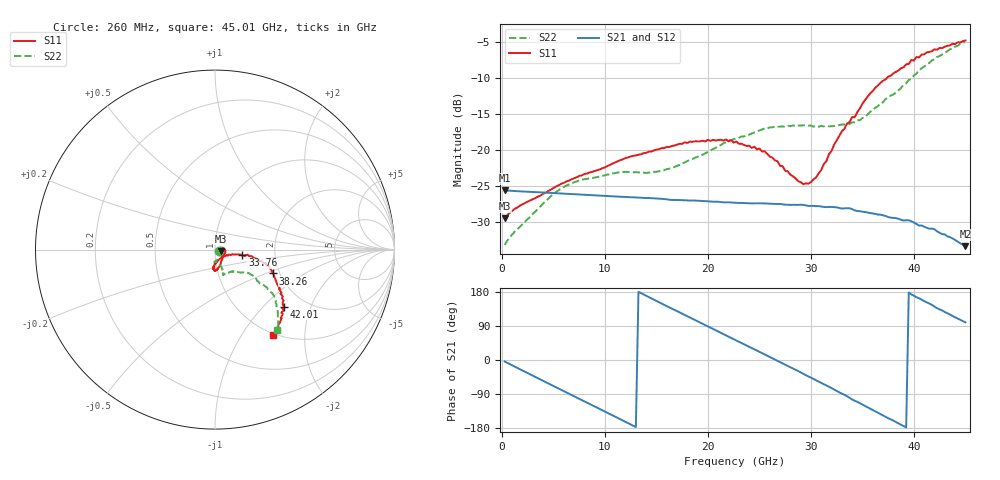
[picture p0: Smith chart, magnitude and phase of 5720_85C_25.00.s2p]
! Device:  ADRF5720
! Description: 0.5dB LSB GaAs MMIC 6-bit Digital Attenuator
! Frequency:  0.000009 -  40 GHz
! Ports:
!	RF1	= Port 1
!	RF2	= Port 2
! Vdd:  3.3 Volt
! Vss:  -3.3 Volt
! Control:  0/3.3 Volt
! State:  25.00 dB attenuation
! Data:  The device was measured using G-S-G Probes on a matrix board.
!  Data was collected using an calibrated 4 port network analyzer.
!  The reference plane for this measurement is at the launchers.
! Note:  Analog Devices supplies this data as a sample of measured data
!  for this product.  Your particular data for this product may vary.
!  Data was taken at 85 degrees C.
!  Analog Devices reserves the right to change this data at anytime.
# GHZ S DB R 45.0
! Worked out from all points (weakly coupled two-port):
!   180 points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, 260 MHz to 45.01 GHz, reference 45 ohm
!   highest |S21| = -25.66 dB at 260 MHz (marker M1); lowest = -33.4 dB at 45.01 GHz (marker M2)
!   lowest |S11| = -29.5 dB at 260 MHz (marker M3), VSWR 1.07, Z = 48 - j0.787 ohm
!   |S11| at or under -10 dB: start of sweep to 37.39 GHz
!   |S22| runs from -33.2 to -4.9 dB; largest |S21 - S12| = 0.00029
!   S11 on the Smith chart (normalised r, x): 260 MHz: 1.07, -0.02; 33.76 GHz: 1.36, -0.09; 38.26 GHz: 1.84, -0.56; 42.01 GHz: 1.57, -1.33; 45.01 GHz: 0.97, -1.39
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0.26  -29.52 -14.2  -25.66 -3.8  -25.66 -3.8  -33.25 -22.7
1.26  -28.21 -3.8  -25.75 -17.8  -25.74 -17.7  -31.37 -14.5
4.76  -25.54 -36.0  -26.01 -65.4  -26.00 -65.4  -26.45 -66.1
6.26  -24.41 -45.2  -26.13 -85.7  -26.12 -85.6  -24.98 -76.4
7.76  -23.57 -52.6  -26.25 -105.9  -26.24 -105.8  -24.19 -83.4
11.51  -21.44 -68.3  -26.55 -156.4  -26.54 -156.3  -23.11 -92.8
15.26  -19.92 -78.0  -26.80 152.4  -26.79 152.5  -22.99 -85.3
18.26  -18.86 -84.7  -27.07 112.2  -27.05 112.3  -21.42 -75.3
22.76  -18.86 -92.2  -27.38 51.5  -27.36 51.7  -18.44 -69.8
25.51  -20.21 -93.1  -27.47 14.8  -27.45 15.1  -17.04 -71.9
29.26  -24.78 -59.8  -27.67 -36.4  -27.65 -36.2  -16.60 -71.4
30.26  -24.12 -41.1  -27.81 -49.9  -27.79 -49.6  -16.79 -70.3
31.01  -22.83 -24.1  -27.90 -60.5  -27.88 -60.2  -16.67 -68.0
33.01  -17.44 -11.4  -28.18 -88.6  -28.16 -88.3  -16.49 -58.8
33.76  -16.15 -11.6  -28.14 -99.8  -28.12 -99.5  -16.41 -53.6
35.76  -12.15 -13.3  -28.81 -128.2  -28.79 -127.8  -14.73 -43.6
37.76  -9.70 -19.1  -29.45 -156.7  -29.44 -156.4  -12.45 -35.0
38.26  -9.17 -22.5  -29.51 -163.7  -29.49 -163.3  -12.06 -34.4
39.76  -7.51 -30.9  -29.95 173.3  -29.94 173.6  -10.12 -37.0
42.01  -6.02 -39.5  -31.07 140.9  -31.07 141.2  -7.40 -38.9
43.51  -5.48 -45.8  -32.16 120.0  -32.13 120.3  -6.03 -45.5
45.01  -4.79 -56.1  -33.42 99.4  -33.36 99.9  -4.93 -52.3
